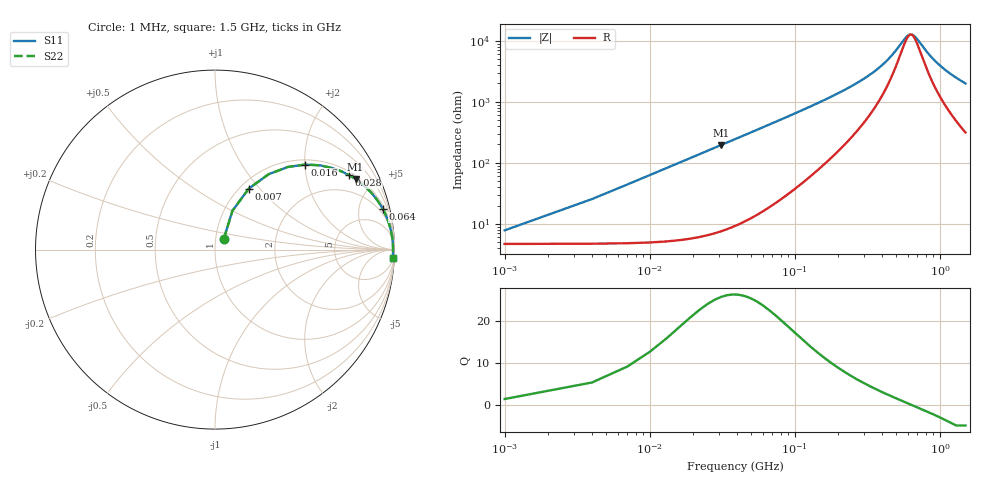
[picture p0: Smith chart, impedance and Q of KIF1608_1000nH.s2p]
# MHz S RI R 50
!Freq ReS11 ImS11 ReS21 ImS21 ReS12 ImS12 ReS22 ImS22
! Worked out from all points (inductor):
!   501 points, 1 MHz to 1.5 GHz, reference 50 ohm
!   read as one part in series: L = 998 nH near 7 MHz
!   highest Q = 25.8 at 31 MHz (marker M1), where L = 1 uH
!   self-resonance near 630.7 MHz
!   S11 on the Smith chart (normalised r, x): 1 MHz: 1.09, +0.13; 7 MHz: 1.10, +0.88; 16 MHz: 1.11, +2.01; 28 MHz: 1.14, +3.52; 64 MHz: 1.35, +8.11; 1.5 GHz: 7, -39
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1  0.0483 0.057  0.9517 -0.057  0.9517 -0.057  0.0483 0.057
7  0.1882 0.3398  0.8118 -0.3398  0.8118 -0.3398  0.1882 0.3398
10  0.2978 0.4194  0.7022 -0.4194  0.7022 -0.4194  0.2978 0.4194
13  0.4061 0.4605  0.5939 -0.4605  0.5939 -0.4605  0.4061 0.4605
16  0.5025 0.4738  0.4975 -0.4738  0.4975 -0.4738  0.5025 0.4738
22  0.6503 0.4553  0.3497 -0.4553  0.3497 -0.4553  0.6503 0.4553
28  0.7477 0.4149  0.2523 -0.4149  0.2523 -0.4149  0.7477 0.4149
31  0.783 0.3933  0.217 -0.3933  0.217 -0.3933  0.783 0.3933
43  0.8711 0.3166  0.1289 -0.3166  0.1289 -0.3166  0.8711 0.3166
64  0.934 0.2275  0.066 -0.2275  0.066 -0.2275  0.934 0.2275
97  0.9666 0.1535  0.0334 -0.1535  0.0334 -0.1535  0.9666 0.1535
136  0.9796 0.1084  0.0204 -0.1084  0.0204 -0.1084  0.9796 0.1084
253  0.9893 0.0518  0.0107 -0.0518  0.0107 -0.0518  0.9893 0.0518
502  0.992 0.0114  0.00798 -0.0114  0.00798 -0.0114  0.992 0.0114
580  0.9921 0.00417  0.00786 -0.00417  0.00786 -0.00417  0.9921 0.00417
625  0.9922 0.00045  0.00784 -0.00045  0.00784 -0.00045  0.9922 0.00045
670  0.9922 -0.00301  0.00784 0.00301  0.00784 0.00301  0.9922 -0.00301
751  0.9921 -0.00872  0.00791 0.00872  0.00791 0.00872  0.9921 -0.00872
868  0.9919 -0.0161  0.00809 0.0161  0.00809 0.0161  0.9919 -0.0161
1003  0.9916 -0.0239  0.00839 0.0239  0.00839 0.0239  0.9916 -0.0239
1252  0.9908 -0.0368  0.00918 0.0368  0.00918 0.0368  0.9908 -0.0368
1500  0.9898 -0.0485  0.0102 0.0485  0.0102 0.0485  0.9898 -0.0485
